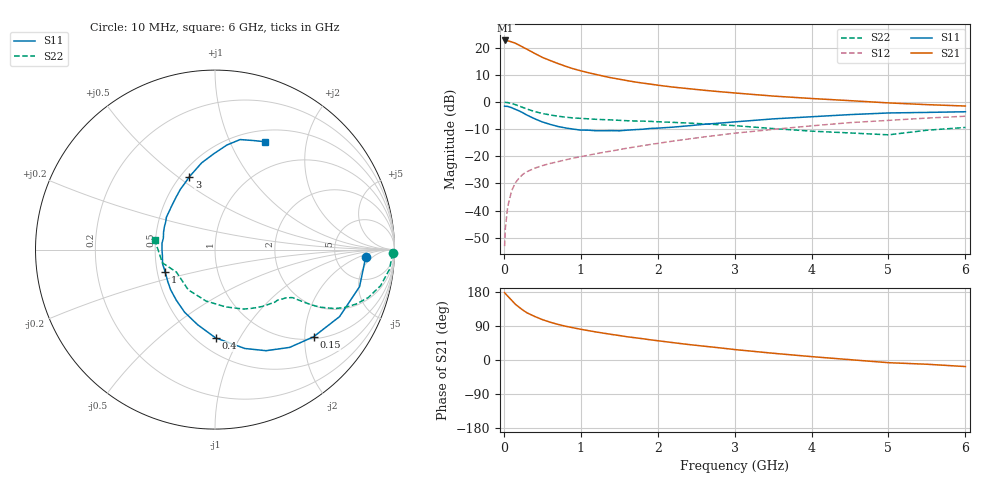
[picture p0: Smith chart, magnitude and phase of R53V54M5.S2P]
! SIEMENS Small Signal Semiconductors
! BFR183
! Si NPN RF Bipolar Junction Transistor in SOT23
! VCE = 3.5 V  IC = 4.5 mA
! Common Emitter S-Parameters:  May  1996
# GHz  S  MA  R  50
!  f  S11  S21  S12  S22
! GHz  MAG  ANG  MAG  ANG  MAG  ANG  MAG  ANG
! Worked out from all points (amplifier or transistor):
!   36 points, 10 MHz to 6 GHz, reference 50 ohm
!   highest |S21| = 22.7 dB at 20 MHz (marker M1)
!   |S21| within 3 dB of that: start of sweep to 283.9 MHz
!   unconditionally stable (mu >= 1): 1.101 GHz to 2.653 GHz
!   at 250 MHz: K = 0.39, MSG = 23.4 dB, |S12| = -26.6 dB
!   at 1.4 GHz: K = 1.06, MAG = 12.0 dB, |S12| = -18.1 dB
!   at 6 GHz: K = 0.88, MSG = 1.9 dB, |S12| = -5.2 dB
!   S11 on the Smith chart (normalised r, x): 10 MHz: 11, -3; 150 MHz: 1.05, -2.21; 400 MHz: 0.61, -0.80; 1 GHz: 0.55, -0.15; 3 GHz: 0.55, +0.55; 6 GHz: 0.64, +1.36
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0.01  0.8401 -3.0  13.46 177.9  0.0022 89.5  0.9912 -1.2
0.02  0.8355 -5.6  13.66 175.3  0.0048 85.3  0.9857 -2.6
0.05  0.8315 -14.4  13.49 168.6  0.0117 81.8  0.9783 -6.5
0.1  0.788 -28.3  12.85 158.0  0.0229 76.1  0.9443 -12.3
0.15  0.7332 -41.5  12.16 147.1  0.0324 69.5  0.8945 -17.4
0.2  0.6857 -52.6  11.18 139.0  0.04 65.4  0.8427 -21.1
0.25  0.631 -63.2  10.24 131.3  0.0469 61.5  0.7921 -24.0
0.3  0.5755 -73.2  9.415 124.6  0.0519 58.9  0.7441 -26.2
0.4  0.4919 -89.6  7.898 115.0  0.0602 55.7  0.668 -28.7
0.5  0.4297 -103.0  6.672 106.6  0.0672 54.2  0.6159 -29.9
0.6  0.3881 -115.8  5.841 99.9  0.0736 54.0  0.5786 -30.5
0.7  0.3552 -127.3  5.157 94.2  0.0793 54.3  0.5493 -31.0
0.8  0.3333 -137.9  4.583 89.2  0.0857 54.7  0.5266 -31.5
1  0.3037 -156.3  3.763 81.1  0.0982 55.9  0.5001 -32.3
1.1  0.3028 -164.9  3.471 77.5  0.1047 56.6  0.4902 -33.3
1.6  0.3028 161.2  2.486 61.4  0.1409 57.9  0.4524 -38.1
2.2  0.3446 133.9  1.886 45.8  0.1908 56.9  0.422 -47.1
3  0.4306 109.3  1.47 27.6  0.2662 51.2  0.3671 -64.5
3.5  0.4893 98.7  1.289 17.8  0.3132 46.0  0.3242 -79.7
4.5  0.5866 83.5  1.061 0.9  0.4173 34.3  0.2691 -123.7
5.5  0.644 70.7  0.896 -11.2  0.5063 21.6  0.3022 -165.9
6  0.662 65.2  0.844 -17.3  0.5475 13.4  0.3398 171.0
